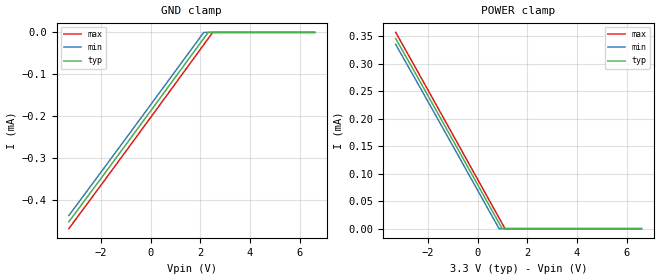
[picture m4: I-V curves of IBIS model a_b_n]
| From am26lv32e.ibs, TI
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[Model]   a_b_n
Model_type   Input
Vinl = 0.8
Vinh = 2.0
|   typ   min   max
|   (nom PVT)   (fast PVT)   (slow PVT)
C_comp   3.305e-12   3.305e-12   3.478e-12
| Where nom  PVT is Nominal Process, 3.3V, 27C
|   Fast PVT is Strong Process,  3.6V, -40C
|   Slow PVT is Weak Process,   3V, 125C
[Voltage Range]   3.3   3   3.6
|Junction Temperature
[Temperature Range]   27   125   -40
[Power Clamp Reference]   3.3   3   3.6
[GND Clamp Reference]   0   0   0
[GND Clamp]
|   Voltage   I(typ)   I(min)   I(max)
-3.3V     -452.9uA   -438.2uA   -469.3uA
2.133V    -14.54uA   -220nA     -29.61uA
2.31V     -177.4nA   0A         -15.2uA
2.502V    0A         0A         0A
6.6V      0A         0A         0A
[POWER Clamp]
|   Voltage   I(typ)   I(min)   I(max)
-3.3V     345.9uA    335.3uA    357.2uA
864mV     10.04uA    22.78nA    19.47uA
986.7mV   90.31nA    0A         9.484uA
1.102V    0A         0A         133nA
6.6V      0A         0A         0A
